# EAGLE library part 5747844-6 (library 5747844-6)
Body Features: Connector Profile Standard | Mating Feature Material Zinc | Assembly Process Feature Material Copper Alloy | Mating Feature Plating Material Clear Chromate | Primary Product Color Black | Shell Plating Material Tin | Insert Material Zinc | Configuration Features: Number of Rows 2 | Number of Positions 9 | PCB Mount Orientation Right Angle | Contact Features: Contact Base Material Phosphor Bronze | Contact Mating Area Plating Material Thickness 30 MICIN | Contact Mating Area Plating Material G Source: Datasheet
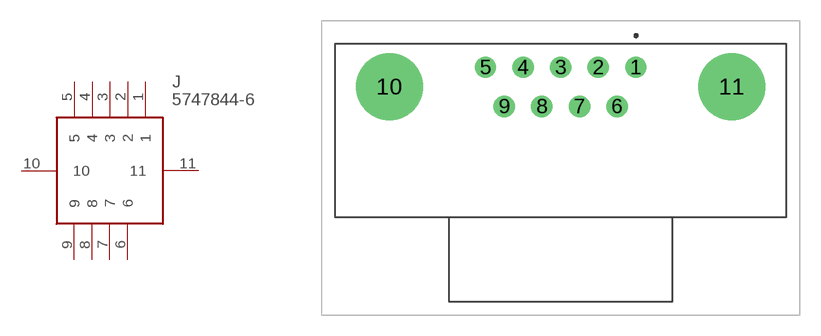
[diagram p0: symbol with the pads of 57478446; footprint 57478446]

Designator prefix J

## 5747844-6 (Description: Body Features: Connector Profile Standard | Mating Feature Material Zinc | Assembly Process Feature Material Copper Alloy | Mating Feature Plating Material Clear Chromate | Primary Product Color Black | Shell Plating Material Tin | Insert Material Zinc | Configuration Features: Number of Rows 2 | Number of Positions 9 | PCB Mount Orientation Right Angle | Contact Features: Contact Base Material Phosphor Bronze | Contact Mating Area Plating Material Thickness 30 MICIN | Contact Mating Area Plating Material G; Height: 12mm; Manufacturer_Name: TE Connectivity; Manufacturer_Part_Number: 5747844-6; Mouser_Part_Number: 571-5747844-6; Mouser_Price-Stock: https://www.mouser.co.uk/ProductDetail/TE-Connectivity/5747844-6?qs=x6EjVpvqMVNBaI3EeeZZVw%3D%3D)  [57478446]
1  1
2  2
3  3
4  4
5  5
6  6
7  7
8  8
9  9
10  10
11  11

## Footprint 57478446 (pad centres in mm)
5747844-6
drill 1.041 pad 1.562: 1 5.486,7.344; 2 2.743,7.344; 3 0,7.344; 4 -2.743,7.344; 5 -5.486,7.344; 6 4.115,4.499; 7 1.372,4.499; 8 -1.372,4.499; 9 -4.115,4.499
drill 3.251 pad 4.877: 10 -12.497,5.921; 11 12.497,5.921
